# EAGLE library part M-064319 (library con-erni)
50 pol. male SMC CONNECTOR vertical , type Q, low profile Source: http://www.erni.com/DB/PDF-Drawing/SMC/064319.pdf
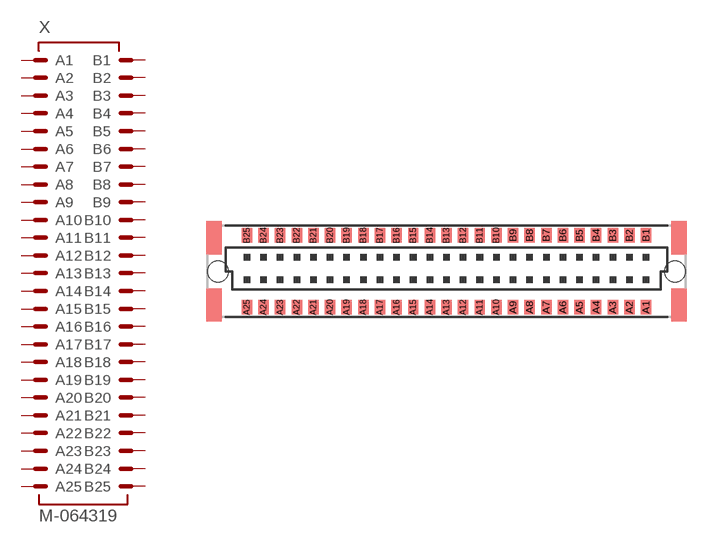
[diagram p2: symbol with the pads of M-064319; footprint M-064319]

Designator prefix X

## M-064319 (OC_FARNELL: unknown; OC_NEWARK: unknown)  [M-064319]
A1  A1  pas
A2  A2  pas
A3  A3  pas
A4  A4  pas
A5  A5  pas
A6  A6  pas
A7  A7  pas
A8  A8  pas
A9  A9  pas
A10  A10  pas
A11  A11  pas
A12  A12  pas
A13  A13  pas
A14  A14  pas
A15  A15  pas
A16  A16  pas
A17  A17  pas
A18  A18  pas
A19  A19  pas
A20  A20  pas
A21  A21  pas
A22  A22  pas
A23  A23  pas
A24  A24  pas
A25  A25  pas
B1  B1  pas
B2  B2  pas
B3  B3  pas
B4  B4  pas
B5  B5  pas
B6  B6  pas
B7  B7  pas
B8  B8  pas
B9  B9  pas
B10  B10  pas
B11  B11  pas
B12  B12  pas
B13  B13  pas
B14  B14  pas
B15  B15  pas
B16  B16  pas
B17  B17  pas
B18  B18  pas
B19  B19  pas
B20  B20  pas
B21  B21  pas
B22  B22  pas
B23  B23  pas
B24  B24  pas
B25  B25  pas

## Footprint M-064319 (pad centres in mm)
50 pol. male SMC CONNECTOR vertical , type Q, low profile Source: http://www.erni.com/DB/PDF-Drawing/SMC/064319.pdf
smd 0.8 x 1.1: A1 15.24,-2.75; A2 13.97,-2.75; A3 12.7,-2.75; A4 11.43,-2.75; A5 10.16,-2.75; A6 8.89,-2.75; A7 7.62,-2.75; A8 6.35,-2.75; A9 5.08,-2.75; A10 3.81,-2.75; A11 2.54,-2.75; A12 1.27,-2.75; A13 0,-2.75; A14 -1.27,-2.75; A15 -2.54,-2.75; A16 -3.81,-2.75; A17 -5.08,-2.75; A18 -6.35,-2.75; A19 -7.62,-2.75; A20 -8.89,-2.75; A21 -10.16,-2.75; A22 -11.43,-2.75; A23 -12.7,-2.75; A24 -13.97,-2.75; A25 -15.24,-2.75; B1 15.24,2.75; B2 13.97,2.75; B3 12.7,2.75; B4 11.43,2.75; B5 10.16,2.75; B6 8.89,2.75; B7 7.62,2.75; B8 6.35,2.75; B9 5.08,2.75; B10 3.81,2.75; B11 2.54,2.75; B12 1.27,2.75; B13 0,2.75; B14 -1.27,2.75; B15 -2.54,2.75; B16 -3.81,2.75; B17 -5.08,2.75; B18 -6.35,2.75; B19 -7.62,2.75; B20 -8.89,2.75; B21 -10.16,2.75; B22 -11.43,2.75; B23 -12.7,2.75; B24 -13.97,2.75; B25 -15.24,2.75
hole 1.6 at 17.45,0
hole 1.6 at -17.45,0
